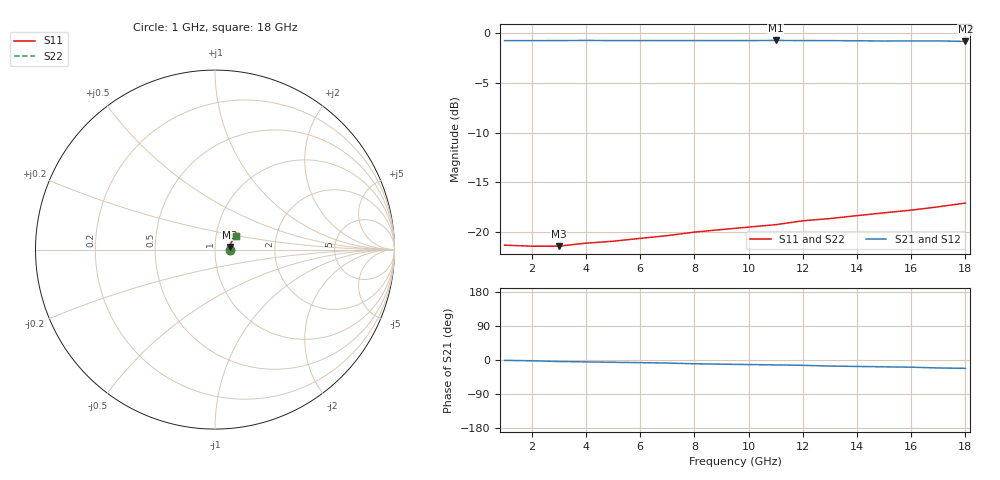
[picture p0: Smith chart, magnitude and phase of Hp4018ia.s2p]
!HPND-4018 beam lead PIN diode
!Series configuration S-parameters If=1mA.  Last updated 10/3/97
# mhz s ma r 50
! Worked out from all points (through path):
!   18 points, 1 GHz to 18 GHz, reference 50 ohm
!   highest |S21| = -0.73 dB at 11 GHz (marker M1); lowest = -0.8 dB at 18 GHz (marker M2)
!   group delay of S21, straight-line fit = 3.39 ps
!   lowest |S11| = -21.4 dB at 3 GHz (marker M3), VSWR 1.19, Z = 59.1 + j1.76 ohm
!   |S11| at or under -10 dB: start of sweep to end of sweep
!   |S22| runs from -21.4 to -17.1 dB; largest |S21 - S12| = 0
1000  0.086 -1.0  0.917 -1.0  0.917 -1.0  0.086 -1.0
2000  0.085 5.0  0.917 -2.0  0.917 -2.0  0.085 5.0
3000  0.085 10.0  0.918 -4.0  0.918 -4.0  0.085 10.0
4000  0.088 14.0  0.919 -5.0  0.919 -5.0  0.088 14.0
5000  0.09 18.0  0.918 -6.0  0.918 -6.0  0.09 18.0
6000  0.093 20.0  0.918 -7.0  0.918 -7.0  0.093 20.0
7000  0.096 22.0  0.918 -8.0  0.918 -8.0  0.096 22.0
8000  0.1 24.0  0.918 -10.0  0.918 -10.0  0.1 24.0
9000  0.103 26.0  0.918 -11.0  0.918 -11.0  0.103 26.0
10000  0.106 27.0  0.918 -12.0  0.918 -12.0  0.106 27.0
11000  0.109 28.0  0.919 -13.0  0.919 -13.0  0.109 28.0
12000  0.114 28.0  0.918 -14.0  0.918 -14.0  0.114 28.0
13000  0.117 29.0  0.917 -16.0  0.917 -16.0  0.117 29.0
14000  0.121 30.0  0.916 -17.0  0.916 -17.0  0.121 30.0
15000  0.125 30.0  0.913 -18.0  0.913 -18.0  0.125 30.0
16000  0.129 31.0  0.914 -19.0  0.914 -19.0  0.129 31.0
17000  0.134 31.0  0.914 -21.0  0.914 -21.0  0.134 31.0
18000  0.14 32.0  0.909 -22.0  0.909 -22.0  0.14 32.0
